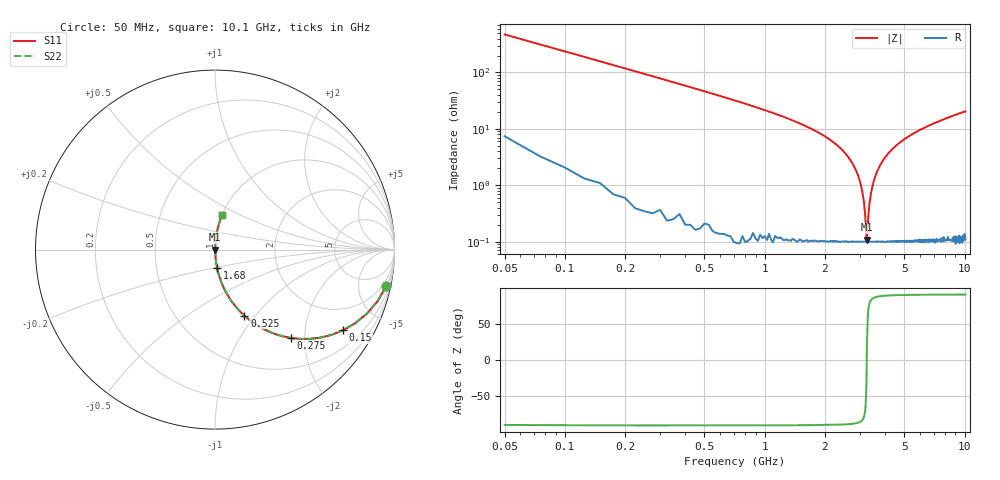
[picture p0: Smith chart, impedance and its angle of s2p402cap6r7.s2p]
! AVX Thin Film Operation		Date: April 2003
! Description: Accu-P® Series, Thin Film, SMD, RF Capacitor
! Part Number: 04025J6R7BBS
! 50 MHz  -  10.05 GHz
! Serial Measurements
# hz S db R 50
!	S11		S21		S12		S22
!	dB	Phase	dB	Phase	dB	Phase	dB	Phase
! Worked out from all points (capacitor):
!   400 points, 50 MHz to 10.1 GHz, reference 50 ohm
!   read as one part in series: C = 6.7 pF near 100 MHz
!   lowest |Z| = 109 mohm at 3.25 GHz (marker M1)
!   series resonance near 3.243 GHz, so ESL is about 360 pH
!   S11 on the Smith chart (normalised r, x): 50 MHz: 1.14, -9.46; 150 MHz: 1.02, -3.16; 275 MHz: 1.01, -1.71; 525 MHz: 1.00, -0.88; 1.68 GHz: 1.00, -0.21; 10.1 GHz: 1.00, +0.41
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5e7  -0.22 -11.9  -13.70 77.2  -13.70 77.2  -0.22 -11.9
1e8  -0.74 -22.8  -8.24 66.7  -8.24 66.7  -0.74 -22.8
1.5e8  -1.49 -32.2  -5.46 57.4  -5.46 57.4  -1.49 -32.2
2.75e8  -3.75 -49.3  -2.41 40.5  -2.41 40.5  -3.75 -49.3
5.25e8  -7.90 -66.0  -0.78 23.7  -0.78 23.7  -7.90 -66.0
1.68e9  -19.70 -83.5  -0.06 5.9  -0.06 5.9  -19.70 -83.5
1.73e9  -20.20 -83.8  -0.05 5.6  -0.05 5.6  -20.20 -83.8
2.43e9  -27.30 -86.2  -0.02 2.5  -0.02 2.5  -27.30 -86.2
2.88e9  -35.10 -85.7  -0.01 1.0  -0.01 1.0  -35.10 -85.7
3.03e9  -39.90 -83.8  -0.01 0.6  -0.01 0.6  -39.90 -83.8
3.13e9  -45.30 -79.1  -0.01 0.3  -0.01 0.3  -45.30 -79.1
3.18e9  -50.00 -71.4  -0.01 0.2  -0.01 0.2  -50.00 -71.4
3.23e9  -58.20 -35.3  -0.01 0.0  -0.01 0.0  -58.20 -35.3
3.25e9  -59.30 22.9  -0.01 -0.0  -0.01 -0.0  -59.30 22.9
3.3e9  -50.90 69.3  -0.01 -0.2  -0.01 -0.2  -50.90 69.3
3.4e9  -43.00 81.5  -0.01 -0.4  -0.01 -0.4  -43.00 81.5
3.6e9  -36.20 85.4  -0.01 -0.9  -0.01 -0.9  -36.20 85.4
3.95e9  -30.70 86.4  -0.01 -1.7  -0.01 -1.7  -30.70 86.4
5.08e9  -23.40 85.3  -0.03 -3.9  -0.03 -3.9  -23.40 85.3
6.75e9  -18.70 82.8  -0.07 -6.7  -0.07 -6.7  -18.70 82.8
8.43e9  -15.90 80.4  -0.12 -9.2  -0.12 -9.2  -15.90 80.4
1.01e10  -14.00 78.2  -0.19 -11.5  -0.19 -11.5  -14.00 78.2
